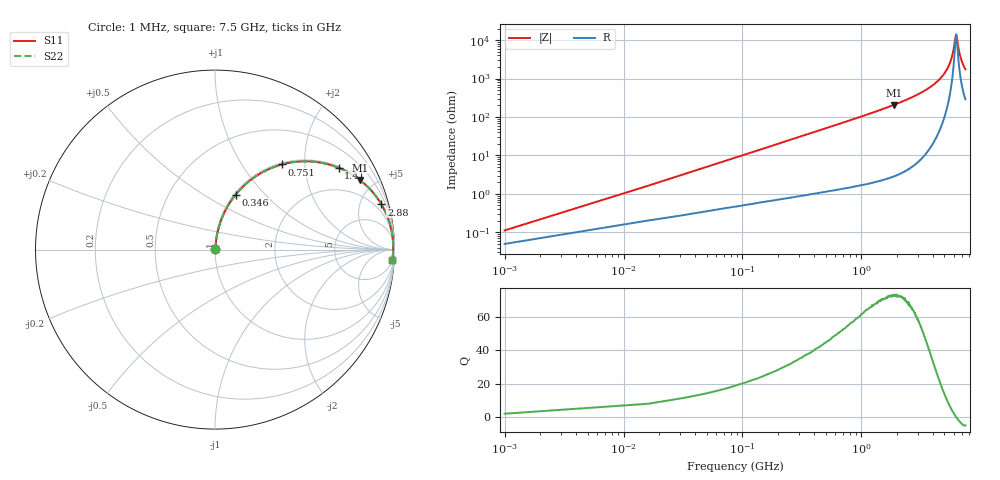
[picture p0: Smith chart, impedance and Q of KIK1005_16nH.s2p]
!version-3
!date-01.2023
!Series
# MHz S RI R 50
!Freq ReS11 ImS11 ReS21 ImS21 ReS12 ImS12 ReS22 ImS22
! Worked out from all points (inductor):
!   501 points, 1 MHz to 7.5 GHz, reference 50 ohm
!   read as one part in series: L = 16 nH near 31 MHz
!   highest Q = 72.7 at 1.88 GHz (marker M1), where L = 17.5 nH
!   self-resonance near 6.27 GHz
!   S11 on the Smith chart (normalised r, x): 1 MHz: 1.00, +0.00; 346 MHz: 1.02, +0.70; 751 MHz: 1.03, +1.53; 1.41 GHz: 1.04, +2.99; 2.88 GHz: 1.12, +7.34; 7.5 GHz: 7, -34
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1  0.000501 0.001  0.9995 -0.001  0.9995 -0.001  0.000501 0.001
46  0.0055 0.0458  0.9945 -0.0458  0.9945 -0.0458  0.0055 0.0458
76  0.0101 0.0753  0.9899 -0.0753  0.9899 -0.0753  0.0101 0.0753
121  0.0198 0.1186  0.9802 -0.1186  0.9802 -0.1186  0.0198 0.1186
181  0.0382 0.174  0.9618 -0.174  0.9618 -0.174  0.0382 0.174
346  0.115 0.3059  0.885 -0.3059  0.885 -0.3059  0.115 0.3059
751  0.3721 0.4742  0.6279 -0.4742  0.6279 -0.4742  0.3721 0.4742
1260  0.6339 0.4743  0.3661 -0.4743  0.3661 -0.4743  0.6339 0.4743
1410  0.6882 0.4561  0.3118 -0.4561  0.3118 -0.4561  0.6882 0.4561
1880  0.8077 0.3873  0.1923 -0.3873  0.1923 -0.3873  0.8077 0.3873
2510  0.8964 0.2975  0.1036 -0.2975  0.1036 -0.2975  0.8964 0.2975
2880  0.9273 0.2515  0.0727 -0.2515  0.0727 -0.2515  0.9273 0.2515
3770  0.9683 0.1628  0.0317 -0.1628  0.0317 -0.1628  0.9683 0.1628
5010  0.9897 0.0708  0.0103 -0.0708  0.0103 -0.0708  0.9897 0.0708
5420  0.9921 0.0462  0.00793 -0.0462  0.00793 -0.0462  0.9921 0.0462
5750  0.993 0.0276  0.00701 -0.0276  0.00701 -0.0276  0.993 0.0276
5960  0.9932 0.0163  0.00683 -0.0163  0.00683 -0.0163  0.9932 0.0163
6260  0.993 0.000986  0.00705 -0.000986  0.00705 -0.000986  0.993 0.000986
6350  0.9928 -0.00347  0.00721 0.00347  0.00721 0.00347  0.9928 -0.00347
6570  0.9922 -0.0143  0.0078 0.0143  0.0078 0.0143  0.9922 -0.0143
6810  0.9913 -0.0255  0.00869 0.0255  0.00869 0.0255  0.9913 -0.0255
7500  0.9875 -0.0554  0.0125 0.0554  0.0125 0.0554  0.9875 -0.0554
